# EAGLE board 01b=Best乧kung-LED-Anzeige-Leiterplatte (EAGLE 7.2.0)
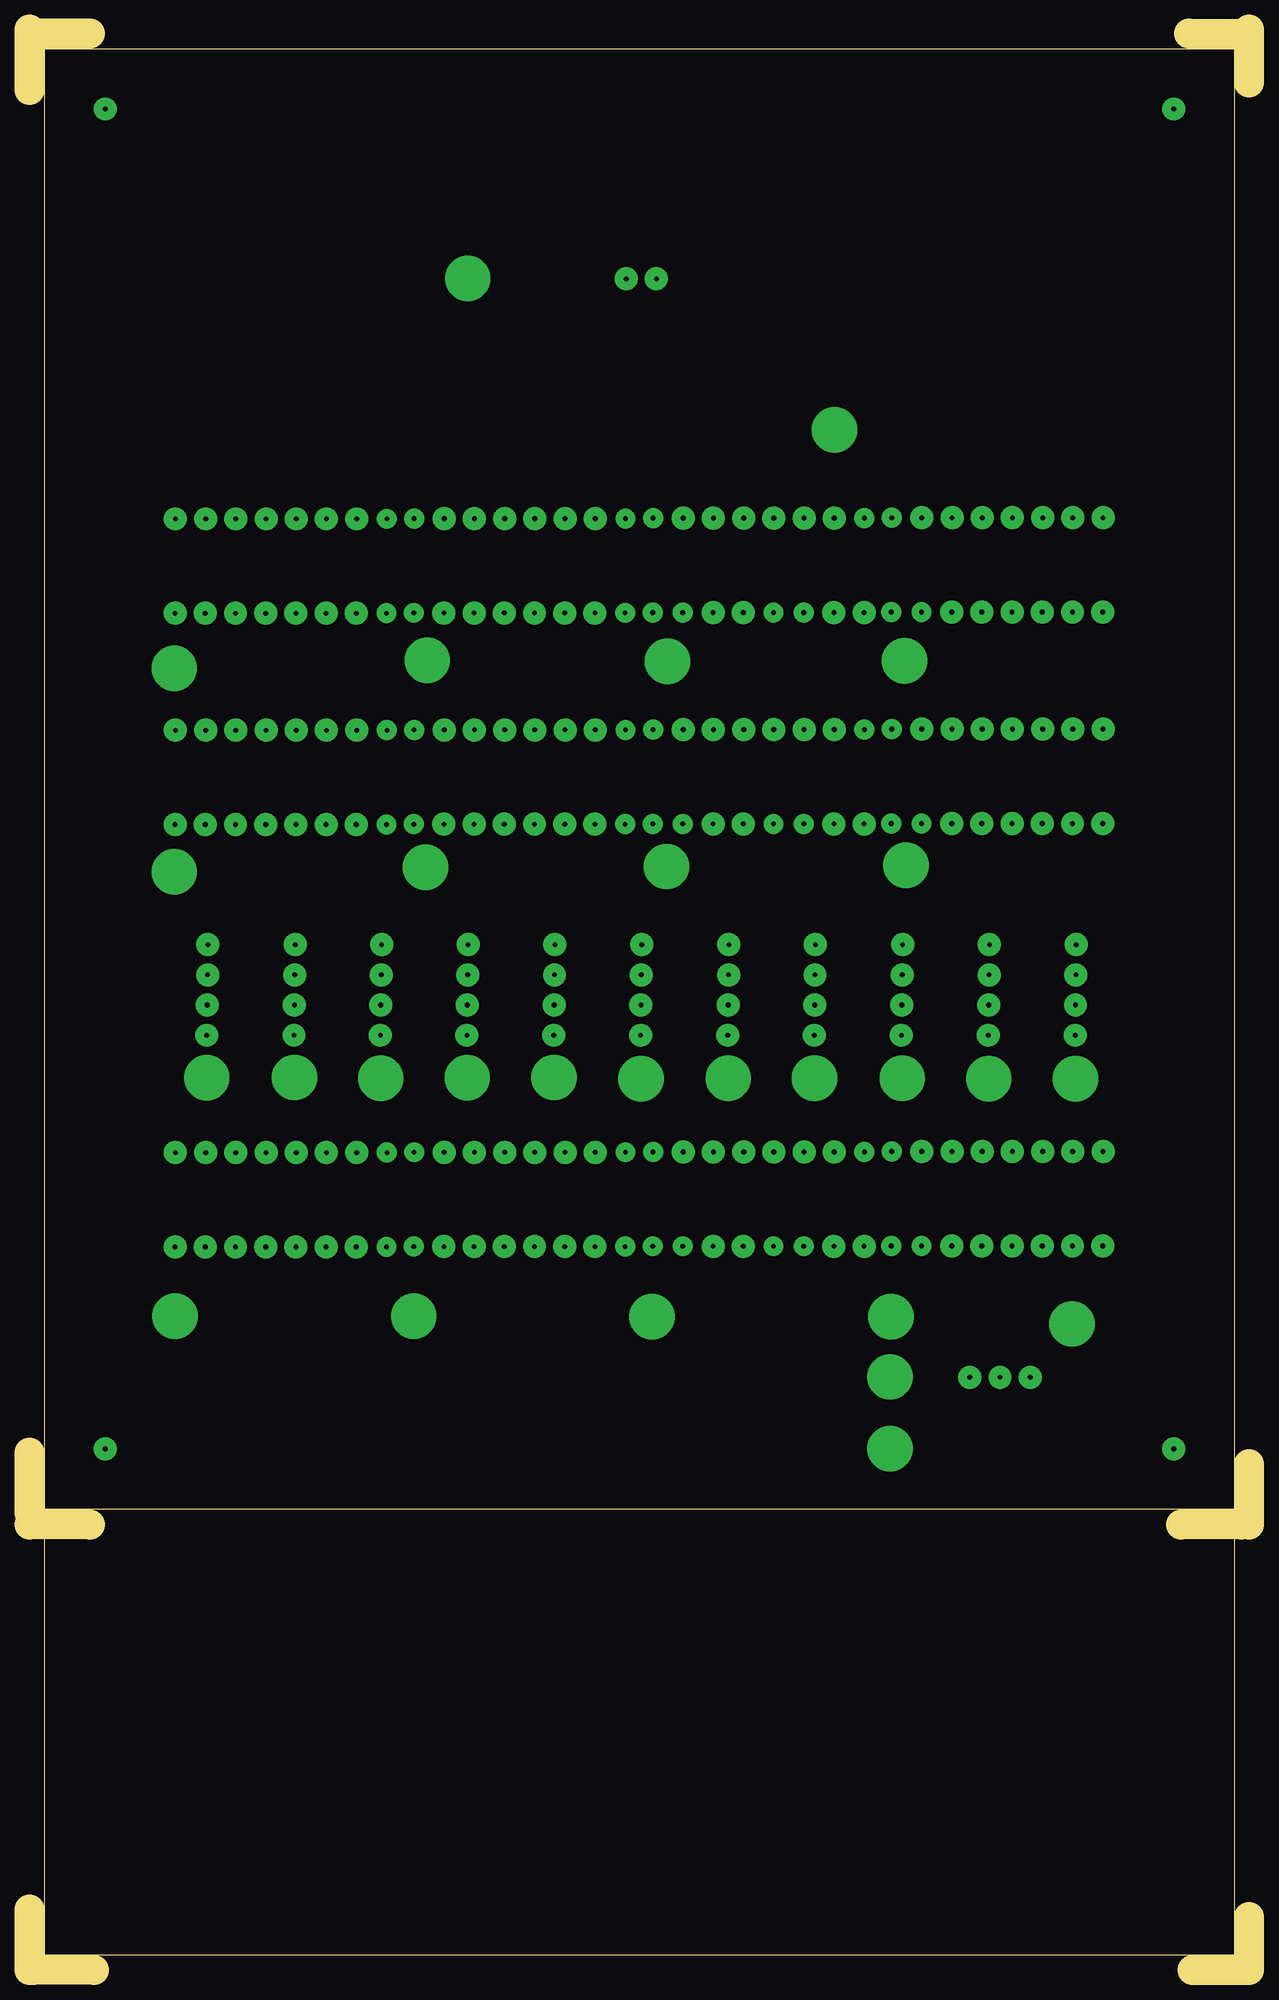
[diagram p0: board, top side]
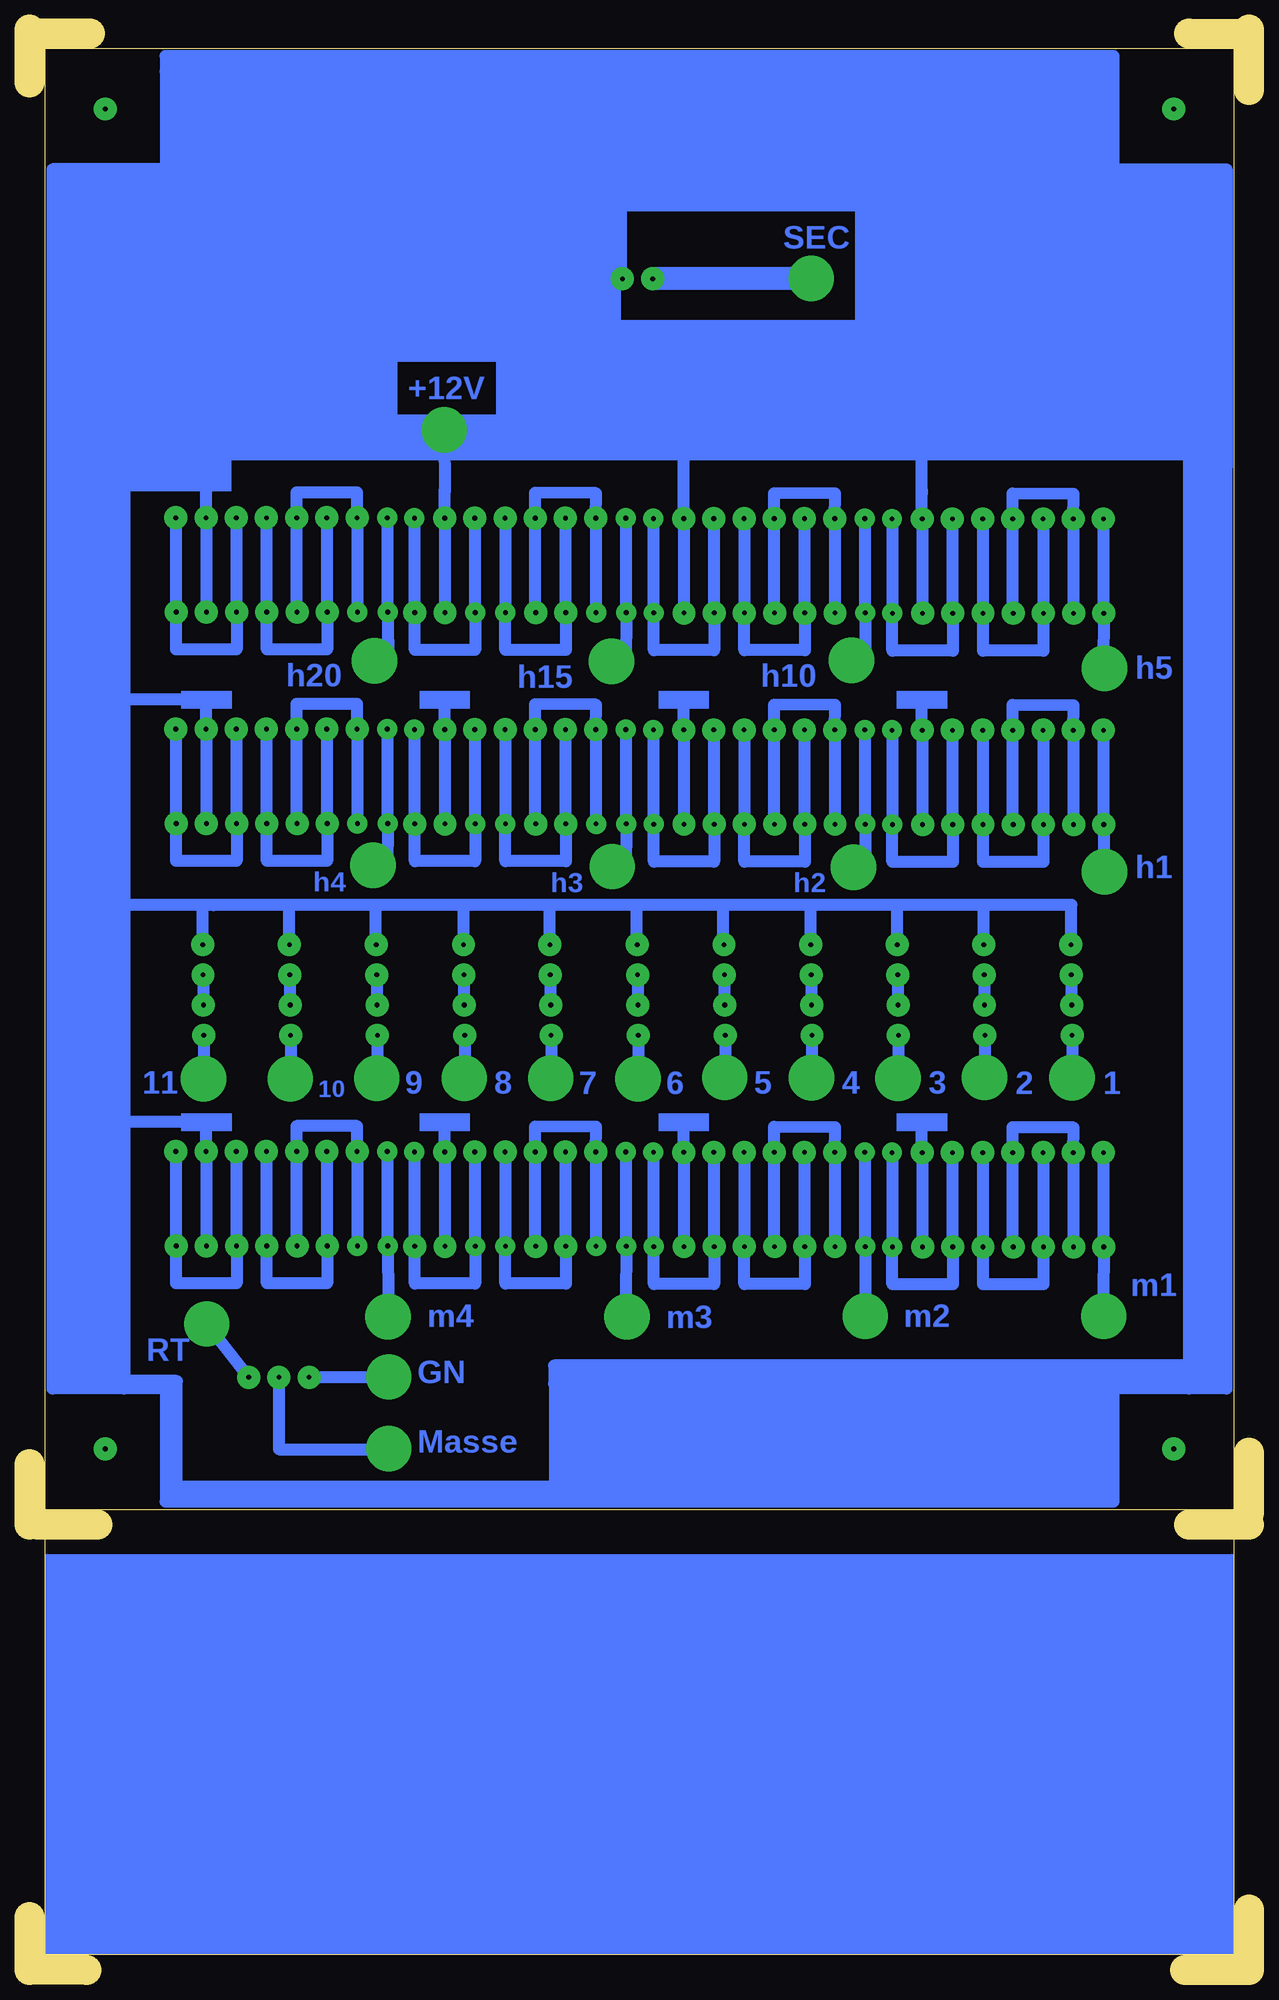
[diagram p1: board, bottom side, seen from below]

Size 102.55 x 163.2 mm. Coordinates in mm from the lower left corner, seen from the top.
Outline: 1.27,38.74 1.27,1.27 101.28,1.27 101.28,38.74
Outline: 1.27,38.74 1.27,161.61 101.28,161.61 101.28,38.74
Outline: 5.4,0 0.32,0
Outline: 0,0 0,5.08
Outline: 97.79,0 102.55,0 102.55,4.45
Outline: 5.08,162.88 0,162.88
Outline: 0,158.12 0,162.88
Outline: 0,162.88 0,163.2
Outline: 102.55,158.75 102.55,163.2
Outline: 97.47,162.88 102.23,162.88
Outline: 101.28,38.74 1.27,38.74
Outline: 0,38.42 0,43.5
Outline: 5.08,37.47 0,37.47
Outline: 101.92,37.47 96.84,37.47
Outline: 102.55,37.47 102.55,42.55
Copper layers (1*16): Top 0.035mm / dielectric 1.5mm / Bottom 0.035mm
Design rules "default": minimum track width 10mil, minimum drill 24mil, track to track 8mil, track to pad 8mil, pad to pad 8mil, via to via 8mil, smd to smd 8mil, copper to edge 40mil, drill to drill 8mil, minimum pad ring 10mil, minimum via ring 8mil, stop-mask expansion 4mil, vias tented up to drill 0mil, thermal gap 10mil

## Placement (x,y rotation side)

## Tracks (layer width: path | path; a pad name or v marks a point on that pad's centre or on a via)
S$1  (via drill 0.4 pad 1.93)
  other vias: 81.6,49.85
S$2  (via drill 0.4 pad 1.93)
  other vias: 96.2,43.82
S$3  (via drill 0 pad 3.81, 0.4 pad 1.93)
  Bottom 1.016: v84.14,49.85 87.63,54.29 v87.66,54.32
S$4  (via drill 0.4 pad 1.93)
  other vias: 6.35,43.82
S$5  (via drill 0 pad 3.81, 0.4 pad 1.93)
  Bottom 1.016: v72.36,49.88 72.39,49.85 v79.06,49.85
  other vias: 72.36,43.85 36.83,142.27 67.69,129.54 33.43,110.14 12.16,109.47 53.63,110.08 73.56,110.11
S$6  (via drill 0.4 pad 1.93)
  other vias: 6.35,156.53
S$7  (via drill 0.4 pad 1.93)
  other vias: 52.71,142.24
S$8  (via drill 0.4 pad 1.93)
  other vias: 50.17,142.24
S$9  (via drill 0.4 pad 1.93)
  other vias: 96.2,156.53
S$10  (via drill 0.4 pad 1.68)
  Bottom 1.016: v32.29,60.83 32.29,56.71
S$11  (via drill 0.4 pad 1.93)
  other vias: 34.83,60.83
S$12  (via drill 0.4 pad 1.93)
  other vias: 42.45,60.83
S$13  (via drill 0.4 pad 1.68, 0.4 pad 1.93)
  Bottom 1.016: v44.99,60.83 44.99,57.69 50.07,57.69 v50.07,60.83
S$14  (via drill 0.4 pad 1.93)
  other vias: 47.53,60.83
S$15  (via drill 0.4 pad 1.68)
  other vias: 32.32,68.77
S$16  (via drill 0.4 pad 1.93)
  Bottom 1.016: 34.86,60.74 v34.86,68.77 34.83,70.87 39.97,70.9 39.97,60.83
S$17  (via drill 0.4 pad 1.93)
  Bottom 1.016: v37.37,60.83 37.37,60.8 | 37.37,60.74 37.37,57.69 42.45,57.69 42.45,60.8 | v37.4,68.77 37.4,60.8 37.37,60.8 | 37.37,60.8 37.37,60.74 | 37.37,60.74 37.43,60.74
S$18  (via drill 0.4 pad 1.93)
  other vias: 39.94,68.77
S$19  (via drill 0.4 pad 1.93)
  Bottom 1.016: v42.48,68.77 42.48,60.8
S$20  (via drill 0.4 pad 1.93)
  Bottom 1.016: v45.02,68.77 45.02,60.8
S$21  (via drill 0.4 pad 1.93)
  Bottom 1.016: v47.56,68.77 47.56,60.8
S$22  (via drill 0.4 pad 1.68)
  Bottom 1.016: v50.1,68.77 50.1,60.83
S$23  (via drill 0.4 pad 1.93)
  other vias: 39.91,60.83
S$24
  Bottom 1.016: 32.32,68.71 32.32,60.83
S$25  (via drill 0.4 pad 1.68)
  Bottom 1.016: v52.39,60.87 52.42,56.39
S$26  (via drill 0.4 pad 1.68)
  other vias: 54.93,60.86
S$27  (via drill 0.4 pad 1.68)
  other vias: 62.55,60.86
S$28  (via drill 0.4 pad 1.68, 0.4 pad 1.93)
  Bottom 1.016: v65.09,60.87 65.09,57.72 70.17,57.72 v70.17,60.87
S$29  (via drill 0.4 pad 1.93)
  other vias: 67.63,60.86
S$30  (via drill 0.4 pad 1.68)
  other vias: 52.42,68.8
S$31  (via drill 0.4 pad 1.93)
  Bottom 1.016: 54.96,60.77 v54.96,68.8 54.93,70.9 60.07,70.93 60.07,60.87
S$32  (via drill 0.4 pad 1.93)
  Bottom 1.016: v57.47,60.87 57.47,60.83 | 57.47,60.77 57.47,57.72 62.55,57.72 62.55,60.83 | v57.5,68.8 57.5,60.83 57.47,60.83 | 57.47,60.83 57.47,60.77 | 57.47,60.77 57.53,60.77
S$33  (via drill 0.4 pad 1.93)
  other vias: 60.04,68.8
S$34  (via drill 0.4 pad 1.93)
  Bottom 1.016: v62.58,68.8 62.58,60.83
S$35  (via drill 0.4 pad 1.93)
  Bottom 1.016: v65.12,68.8 65.12,60.83
S$36  (via drill 0.4 pad 1.93)
  Bottom 1.016: v67.66,68.8 67.66,60.83
S$37  (via drill 0.4 pad 1.68)
  Bottom 1.016: v70.2,68.8 70.2,60.87
S$38  (via drill 0.4 pad 1.93)
  other vias: 60.01,60.86
S$39
  Bottom 1.016: 52.42,68.74 52.42,60.87
S$40  (via drill 0.4 pad 1.68)
  Bottom 1.016: v72.45,60.9 72.42,56.32
S$41  (via drill 0.4 pad 1.68)
  other vias: 74.99,60.9
S$42  (via drill 0.4 pad 1.93)
  other vias: 82.61,60.9
S$43  (via drill 0.4 pad 1.93)
  Bottom 1.016: v85.15,60.9 85.15,57.75 90.23,57.75 v90.23,60.9
S$44  (via drill 0.4 pad 1.93)
  other vias: 87.69,60.9
S$45  (via drill 0.4 pad 1.68)
  other vias: 72.49,68.83
S$46  (via drill 0.4 pad 1.93)
  Bottom 1.016: 75.02,60.8 v75.02,68.83 75.02,70.96 80.14,70.96 80.14,60.9
S$47  (via drill 0.4 pad 1.93)
  Bottom 1.016: v77.53,60.9 77.53,60.87 | 77.53,60.8 77.53,57.75 82.61,57.75 82.61,60.87 | v77.56,68.83 77.56,60.87 77.53,60.87 | 77.53,60.87 77.53,60.8 | 77.53,60.8 77.6,60.8
S$48  (via drill 0.4 pad 1.93)
  other vias: 80.11,68.83
S$49  (via drill 0.4 pad 1.93)
  Bottom 1.016: v82.64,68.83 82.64,60.87
S$50  (via drill 0.4 pad 1.93)
  Bottom 1.016: v85.19,68.83 85.19,60.87
S$51  (via drill 0.4 pad 1.93)
  Bottom 1.016: v87.72,68.83 87.72,60.87
S$52  (via drill 0.4 pad 1.93)
  Bottom 1.016: v90.27,68.83 90.27,60.9
S$53  (via drill 0.4 pad 1.93)
  other vias: 80.07,60.9
S$54
  Bottom 1.016: 72.48,68.77 72.48,60.9
S$55
  Bottom 1.016: 27.53,68.74 27.53,71.12
S$56
  Bottom 1.016: 47.56,68.74 47.56,71.12
S$57
  Bottom 1.016: 67.66,68.74 67.66,71.12
S$58
  Bottom 1.016: 87.69,68.74 87.69,71.12
S$59
  Bottom 1.016: 88.93,71.31 96.01,71.31 96.01,71.34
S$60  (via drill 0.4 pad 1.93)
  Bottom 1.016: v12.22,96.33 12.26,91.92
S$61  (via drill 0.4 pad 1.93)
  other vias: 14.76,96.33
S$62  (via drill 0.4 pad 1.93)
  other vias: 22.38,96.33
S$63  (via drill 0.4 pad 1.68, 0.4 pad 1.93)
  Bottom 1.016: v24.92,96.33 24.92,93.19 30,93.19 v30,96.33
S$64  (via drill 0.4 pad 1.93)
  Bottom 1.016: v12.22,60.8 12.26,56.39
S$65  (via drill 0.4 pad 1.93)
  other vias: 14.76,60.8
S$66  (via drill 0.4 pad 1.93)
  other vias: 22.38,60.8
S$67  (via drill 0.4 pad 1.68, 0.4 pad 1.93)
  Bottom 1.016: v24.92,60.8 24.92,57.66 30,57.66 v30,60.8
S$68  (via drill 0.4 pad 1.93)
  other vias: 27.46,60.8
S$69
  Bottom 1.016: 12.26,68.67 12.26,60.8
S$70  (via drill 0.4 pad 1.93)
  other vias: 12.26,68.74
S$71  (via drill 0.4 pad 1.93)
  Bottom 1.016: 14.79,60.71 v14.79,68.74 14.76,70.83 19.91,70.87 19.91,60.8
S$72  (via drill 0.4 pad 1.93)
  other vias: 19.84,60.8
S$73  (via drill 0.4 pad 1.93)
  other vias: 19.88,68.74
S$74  (via drill 0.4 pad 1.93)
  Bottom 1.016: v22.41,68.74 22.41,60.77
S$75  (via drill 0.4 pad 1.93)
  Bottom 1.016: v24.96,68.74 24.96,60.77
S$76  (via drill 0.4 pad 1.93)
  Bottom 1.016: v27.5,68.74 27.5,60.77
S$77  (via drill 0.4 pad 1.68)
  Bottom 1.016: v30.04,68.74 30.04,60.8
S$78  (via drill 0.4 pad 1.93)
  other vias: 27.46,96.33
S$79  (via drill 0.4 pad 1.93)
  other vias: 12.26,104.27
S$80  (via drill 0.4 pad 1.93)
  Bottom 1.016: 14.79,96.23 v14.79,104.27 14.76,106.36 19.91,106.39 19.91,96.33
S$81  (via drill 0.4 pad 1.93)
  Bottom 1.016: v17.3,60.8 17.3,60.77 | 17.3,60.71 17.3,57.66 22.38,57.66 22.38,60.77 | v17.34,68.74 17.34,60.77 17.3,60.77 | 17.3,60.77 17.3,60.71 | 17.3,60.71 17.37,60.71
S$82  (via drill 0.4 pad 1.93)
  Bottom 1.016: v17.3,96.33 17.3,96.3 | 17.3,96.23 17.3,93.19 22.38,93.19 22.38,96.3 | v17.34,104.27 17.34,96.3 17.3,96.3 | 17.3,96.3 17.3,96.23 | 17.3,96.23 17.37,96.23
S$83  (via drill 0.4 pad 1.93)
  other vias: 19.88,104.27
S$84  (via drill 0.4 pad 1.93)
  Bottom 1.016: v22.41,104.27 22.41,96.3
S$85  (via drill 0.4 pad 1.93)
  Bottom 1.016: v24.96,104.27 24.96,96.3
S$86  (via drill 0.4 pad 1.93)
  Bottom 1.016: v27.5,104.27 27.5,96.3
S$87  (via drill 0.4 pad 1.68)
  Bottom 1.016: v30.04,104.27 30.04,96.33
S$88  (via drill 0.4 pad 1.93)
  other vias: 19.84,96.33
S$89
  Bottom 1.016: 12.26,104.2 12.26,96.33
S$90  (via drill 0.4 pad 1.68)
  Bottom 1.016: v32.29,96.36 32.29,92.23
S$91  (via drill 0.4 pad 1.93)
  other vias: 34.83,96.36
S$92  (via drill 0.4 pad 1.93)
  other vias: 42.45,96.36
S$93  (via drill 0.4 pad 1.68, 0.4 pad 1.93)
  Bottom 1.016: v44.99,96.36 44.99,93.22 50.07,93.22 v50.07,96.36
S$94  (via drill 0.4 pad 1.93)
  other vias: 47.53,96.36
S$95  (via drill 0.4 pad 1.68)
  other vias: 32.32,104.3
S$96  (via drill 0.4 pad 1.93)
  Bottom 1.016: 34.86,96.27 v34.86,104.3 34.83,106.39 39.97,106.43 39.97,96.36
S$97  (via drill 0.4 pad 1.93)
  Bottom 1.016: v37.37,96.36 37.37,96.33 | 37.37,96.27 37.37,93.22 42.45,93.22 42.45,96.33 | v37.4,104.3 37.4,96.33 37.37,96.33 | 37.37,96.33 37.37,96.27 | 37.37,96.27 37.43,96.27
S$98  (via drill 0.4 pad 1.93)
  other vias: 39.94,104.3
S$99  (via drill 0.4 pad 1.93)
  Bottom 1.016: v42.48,104.3 42.48,96.33
S$100  (via drill 0.4 pad 1.93)
  Bottom 1.016: v45.02,104.3 45.02,96.33
S$101  (via drill 0.4 pad 1.93)
  Bottom 1.016: v47.56,104.3 47.56,96.33
S$102  (via drill 0.4 pad 1.68)
  Bottom 1.016: v50.1,104.3 50.1,96.36
S$103  (via drill 0.4 pad 1.93)
  other vias: 39.91,96.36
S$104
  Bottom 1.016: 32.32,104.23 32.32,96.36
S$105  (via drill 0.4 pad 1.68)
  Bottom 1.016: v52.39,96.39 52.42,92.39
S$106  (via drill 0.4 pad 1.68)
  other vias: 54.93,96.39
S$107  (via drill 0.4 pad 1.68)
  other vias: 62.55,96.39
S$108  (via drill 0.4 pad 1.68, 0.4 pad 1.93)
  Bottom 1.016: v65.09,96.39 65.09,93.25 70.17,93.25 v70.17,96.39
S$109  (via drill 0.4 pad 1.93)
  other vias: 67.63,96.39
S$110  (via drill 0.4 pad 1.68)
  other vias: 52.42,104.33
S$111  (via drill 0.4 pad 1.93)
  Bottom 1.016: 54.96,96.3 v54.96,104.33 54.93,106.43 60.07,106.46 60.07,96.39
S$112  (via drill 0.4 pad 1.93)
  Bottom 1.016: v57.47,96.39 57.47,96.36 | 57.47,96.3 57.47,93.25 62.55,93.25 62.55,96.36 | v57.5,104.33 57.5,96.36 57.47,96.36 | 57.47,96.36 57.47,96.3 | 57.47,96.3 57.53,96.3
S$113  (via drill 0.4 pad 1.93)
  other vias: 60.04,104.33
S$114  (via drill 0.4 pad 1.93)
  Bottom 1.016: v62.58,104.33 62.58,96.36
S$115  (via drill 0.4 pad 1.93)
  Bottom 1.016: v65.12,104.33 65.12,96.36
S$116  (via drill 0.4 pad 1.93)
  Bottom 1.016: v67.66,104.33 67.66,96.36
S$117  (via drill 0.4 pad 1.68)
  Bottom 1.016: v70.2,104.33 70.2,96.39
S$118  (via drill 0.4 pad 1.93)
  other vias: 60.01,96.39
S$119
  Bottom 1.016: 52.42,104.27 52.42,96.39
S$120  (via drill 0.4 pad 1.68)
  Bottom 1.016: v72.45,96.42 72.48,92.46
S$121  (via drill 0.4 pad 1.68)
  other vias: 74.99,96.42
S$122  (via drill 0.4 pad 1.93)
  other vias: 82.61,96.42
S$123  (via drill 0.4 pad 1.93)
  Bottom 1.016: v85.15,96.42 85.15,93.28 90.23,93.28 v90.23,96.42
S$124  (via drill 0.4 pad 1.93)
  other vias: 87.69,96.42
S$125  (via drill 0.4 pad 1.68)
  other vias: 72.49,104.36
S$126  (via drill 0.4 pad 1.93)
  Bottom 1.016: 75.02,96.33 v75.02,104.36 75.02,106.49 80.14,106.49 80.14,96.42
S$127  (via drill 0.4 pad 1.93)
  Bottom 1.016: v77.53,96.42 77.53,96.39 | 77.53,96.33 77.53,93.28 82.61,93.28 82.61,96.39 | v77.56,104.36 77.56,96.39 77.53,96.39 | 77.53,96.39 77.53,96.33 | 77.53,96.33 77.6,96.33
S$128  (via drill 0.4 pad 1.93)
  other vias: 80.11,104.36
S$129  (via drill 0.4 pad 1.93)
  Bottom 1.016: v82.64,104.36 82.64,96.39
S$130  (via drill 0.4 pad 1.93)
  Bottom 1.016: v85.19,104.36 85.19,96.39
S$131  (via drill 0.4 pad 1.93)
  Bottom 1.016: v87.72,104.36 87.72,96.39
S$132  (via drill 0.4 pad 1.93)
  Bottom 1.016: v90.27,104.36 90.27,96.42
S$133  (via drill 0.4 pad 1.93)
  other vias: 80.07,96.42
S$134
  Bottom 1.016: 72.48,104.3 72.48,96.42
S$135
  Bottom 1.016: 27.53,104.27 27.53,106.65
S$136
  Bottom 1.016: 47.56,104.27 47.56,106.65
S$137
  Bottom 1.016: 67.66,104.27 67.66,106.65
S$138
  Bottom 1.016: 87.69,104.27 87.69,106.65
S$139
  Bottom 1.016: 88.93,106.84 96.01,106.84
S$140
  Bottom 1.016: 4.98,50.83 58.45,50.83 58.45,49.31
S$141  (via drill 0.4 pad 1.93)
  Bottom 1.016: v12.22,114.11 12.26,109.7
S$142  (via drill 0.4 pad 1.93)
  other vias: 14.76,114.11
S$143  (via drill 0.4 pad 1.93)
  other vias: 22.38,114.11
S$144  (via drill 0.4 pad 1.68, 0.4 pad 1.93)
  Bottom 1.016: v24.92,114.11 24.92,110.97 30,110.97 v30,114.11
S$145  (via drill 0.4 pad 1.93)
  other vias: 27.46,114.11
S$146  (via drill 0.4 pad 1.93)
  other vias: 12.26,122.05
S$147  (via drill 0.4 pad 1.93)
  Bottom 1.016: 14.79,114.01 v14.79,122.05 14.76,124.14 19.91,124.17 19.91,114.11
S$148  (via drill 0.4 pad 1.93)
  Bottom 1.016: v17.3,114.11 17.3,114.08 | 17.3,114.01 17.3,110.97 22.38,110.97 22.38,114.08 | v17.34,122.05 17.34,114.08 17.3,114.08 | 17.3,114.08 17.3,114.01 | 17.3,114.01 17.37,114.01
S$149  (via drill 0.4 pad 1.93)
  other vias: 19.88,122.05
S$150  (via drill 0.4 pad 1.93)
  Bottom 1.016: v22.41,122.05 22.41,114.08
S$151  (via drill 0.4 pad 1.93)
  Bottom 1.016: v24.96,122.05 24.96,114.08
S$152  (via drill 0.4 pad 1.93)
  Bottom 1.016: v27.5,122.05 27.5,114.08
S$153  (via drill 0.4 pad 1.68)
  Bottom 1.016: v30.04,122.05 30.04,114.11
S$154  (via drill 0.4 pad 1.93)
  other vias: 19.84,114.11
S$155
  Bottom 1.016: 12.26,121.98 12.26,114.11
S$156  (via drill 0.4 pad 1.68)
  Bottom 1.016: v32.29,114.14 32.29,110.01
S$157  (via drill 0.4 pad 1.93)
  other vias: 34.83,114.14
S$158  (via drill 0.4 pad 1.93)
  other vias: 42.45,114.14
S$159  (via drill 0.4 pad 1.68, 0.4 pad 1.93)
  Bottom 1.016: v44.99,114.14 44.99,111 50.07,111 v50.07,114.14
S$160  (via drill 0.4 pad 1.93)
  other vias: 47.53,114.14
S$161  (via drill 0.4 pad 1.68)
  other vias: 32.32,122.08
S$162  (via drill 0.4 pad 1.93)
  Bottom 1.016: 34.86,114.05 v34.86,122.08 34.83,124.17 39.97,124.21 39.97,114.14
S$163  (via drill 0.4 pad 1.93)
  Bottom 1.016: v37.37,114.14 37.37,114.11 | 37.37,114.05 37.37,111 42.45,111 42.45,114.11 | v37.4,122.08 37.4,114.11 37.37,114.11 | 37.37,114.11 37.37,114.05 | 37.37,114.05 37.43,114.05
S$164  (via drill 0.4 pad 1.93)
  other vias: 39.94,122.08
S$165  (via drill 0.4 pad 1.93)
  Bottom 1.016: v42.48,122.08 42.48,114.11
S$166  (via drill 0.4 pad 1.93)
  Bottom 1.016: v45.02,122.08 45.02,114.11
S$167  (via drill 0.4 pad 1.93)
  Bottom 1.016: v47.56,122.08 47.56,114.11
S$168  (via drill 0.4 pad 1.68)
  Bottom 1.016: v50.1,122.08 50.1,114.14
S$169  (via drill 0.4 pad 1.93)
  other vias: 39.91,114.14
S$170
  Bottom 1.016: 32.32,122.02 32.32,114.14
S$171  (via drill 0.4 pad 1.68)
  Bottom 1.016: v52.39,114.17 52.42,109.7
S$172  (via drill 0.4 pad 1.68)
  other vias: 54.93,114.17
S$173  (via drill 0.4 pad 1.68)
  other vias: 62.55,114.17
S$174  (via drill 0.4 pad 1.68, 0.4 pad 1.93)
  Bottom 1.016: v65.09,114.17 65.09,111.03 70.17,111.03 v70.17,114.17
S$175  (via drill 0.4 pad 1.93)
  other vias: 67.63,114.17
S$176  (via drill 0.4 pad 1.68)
  other vias: 52.42,122.11
S$177  (via drill 0.4 pad 1.93)
  Bottom 1.016: 54.96,114.08 v54.96,122.11 54.93,124.21 60.07,124.24 60.07,114.17
S$178  (via drill 0.4 pad 1.93)
  Bottom 1.016: v57.47,114.17 57.47,114.14 | 57.47,114.08 57.47,111.03 62.55,111.03 62.55,114.14 | v57.5,122.11 57.5,114.14 57.47,114.14 | 57.47,114.14 57.47,114.08 | 57.47,114.08 57.53,114.08
S$179  (via drill 0.4 pad 1.93)
  other vias: 60.04,122.11
S$180  (via drill 0.4 pad 1.93)
  Bottom 1.016: v62.58,122.11 62.58,114.14
S$181  (via drill 0.4 pad 1.93)
  Bottom 1.016: v65.12,122.11 65.12,114.14
S$182  (via drill 0.4 pad 1.93)
  Bottom 1.016: v67.66,122.11 67.66,114.14
S$183  (via drill 0.4 pad 1.68)
  Bottom 1.016: v70.2,122.11 70.2,114.17
S$184  (via drill 0.4 pad 1.93)
  other vias: 60.01,114.17
S$185
  Bottom 1.016: 52.42,122.05 52.42,114.17
S$186  (via drill 0.4 pad 1.68)
  Bottom 1.016: v72.45,114.2 72.42,109.63
S$187  (via drill 0.4 pad 1.68)
  other vias: 74.99,114.2
S$188  (via drill 0.4 pad 1.93)
  other vias: 82.61,114.2
S$189  (via drill 0.4 pad 1.93)
  Bottom 1.016: v85.15,114.2 85.15,111.06 90.23,111.06 v90.23,114.2
S$190  (via drill 0.4 pad 1.93)
  other vias: 87.69,114.2
S$191  (via drill 0.4 pad 1.68)
  other vias: 72.49,122.14
S$192  (via drill 0.4 pad 1.93)
  Bottom 1.016: 75.02,114.11 v75.02,122.14 75.02,124.27 80.14,124.27 80.14,114.2
S$193  (via drill 0.4 pad 1.93)
  Bottom 1.016: v77.53,114.2 77.53,114.17 | 77.53,114.11 77.53,111.06 82.61,111.06 82.61,114.17 | v77.56,122.14 77.56,114.17 77.53,114.17 | 77.53,114.17 77.53,114.11 | 77.53,114.11 77.6,114.11
S$194  (via drill 0.4 pad 1.93)
  other vias: 80.11,122.14
S$195  (via drill 0.4 pad 1.93)
  Bottom 1.016: v82.64,122.14 82.64,114.17
S$196  (via drill 0.4 pad 1.93)
  Bottom 1.016: v85.19,122.14 85.19,114.17
S$197  (via drill 0.4 pad 1.93)
  Bottom 1.016: v87.72,122.14 87.72,114.17
S$198  (via drill 0.4 pad 1.93)
  Bottom 1.016: v90.27,122.14 90.27,114.2
S$199  (via drill 0.4 pad 1.93)
  other vias: 80.07,114.2
S$200
  Bottom 1.016: 72.48,122.08 72.48,114.2
S$201
  Bottom 1.016: 27.53,122.05 27.53,124.17 27.53,124.43 27.53,128.81
S$202
  Bottom 1.016: 47.56,122.05 47.56,124.43
S$203
  Bottom 1.016: 67.66,122.05 67.66,124.43
S$204
  Bottom 1.016: 87.69,122.05 87.69,124.43
S$205
  Bottom 1.016: 86.14,125.89 96.39,125.79
S$206
  Bottom 1.016: 47.56,124.49 47.56,127.06 47.53,127.06
S$207
  Bottom 1.016: 2.57,126.46 2.57,126.36 2.41,126.36
S$226  (via drill 0.4 pad 1.93)
  other vias: 14.89,78.61
S$227  (via drill 0.4 pad 1.93)
  other vias: 14.92,81.15
S$228  (via drill 0.4 pad 1.93)
  Bottom 1.016: v14.95,83.69 14.95,81.12 14.92,81.12
S$229  (via drill 0.4 pad 1.93)
  other vias: 14.99,86.23
S$230  (via drill 0.4 pad 1.93)
  other vias: 22.22,78.61
S$231  (via drill 0.4 pad 1.93)
  other vias: 22.26,81.15
S$232  (via drill 0.4 pad 1.93)
  Bottom 1.016: v22.29,83.69 22.29,81.12 22.26,81.12
S$233  (via drill 0.4 pad 1.93)
  Bottom 1.016: 14.95,86.23 14.95,89.57 22.32,89.57 | 88.04,86.2 88.04,89.57 22.38,89.57 22.32,89.57 | v22.32,86.23 22.32,89.57
S$234  (via drill 0.4 pad 1.93)
  Bottom 1.016: v29.5,78.61 29.5,74.93
S$235  (via drill 0.4 pad 1.93)
  other vias: 29.53,81.15
S$236  (via drill 0.4 pad 1.93)
  Bottom 1.016: v29.56,83.69 29.56,81.12 29.53,81.12
S$237  (via drill 0.4 pad 1.93)
  Bottom 1.016: v29.59,86.23 29.59,89.44
S$238  (via drill 0.4 pad 1.93)
  other vias: 36.77,78.61
S$239  (via drill 0.4 pad 1.93)
  other vias: 36.8,81.15
S$240  (via drill 0.4 pad 1.93)
  Bottom 1.016: v36.83,83.69 36.83,81.12 36.8,81.12
S$241  (via drill 0.4 pad 1.93)
  other vias: 36.86,86.23
S$242  (via drill 0.4 pad 1.93)
  other vias: 44.07,78.61
S$243  (via drill 0.4 pad 1.93)
  other vias: 44.1,81.15
S$244  (via drill 0.4 pad 1.93)
  Bottom 1.016: v44.13,83.69 44.13,81.12 44.1,81.12
S$245  (via drill 0.4 pad 1.93)
  other vias: 44.16,86.23
S$246  (via drill 0.4 pad 1.93)
  other vias: 51.37,78.61
S$247  (via drill 0.4 pad 1.93)
  other vias: 51.4,81.15
S$248  (via drill 0.4 pad 1.93)
  Bottom 1.016: v51.44,83.69 51.44,81.12 51.4,81.12
S$249  (via drill 0.4 pad 1.93)
  other vias: 51.47,86.23
S$250  (via drill 0.4 pad 1.93)
  other vias: 58.71,78.61
S$251  (via drill 0.4 pad 1.93)
  other vias: 58.74,81.15
S$252  (via drill 0.4 pad 1.93)
  Bottom 1.016: v58.77,83.69 58.77,81.12 58.74,81.12
S$253  (via drill 0.4 pad 1.93)
  other vias: 58.8,86.23
S$254  (via drill 0.4 pad 1.93)
  other vias: 65.98,78.61
S$255  (via drill 0.4 pad 1.93)
  other vias: 66.01,81.15
S$256  (via drill 0.4 pad 1.93)
  Bottom 1.016: v66.04,83.69 66.04,81.12 66.01,81.12
S$257  (via drill 0.4 pad 1.93)
  Bottom 1.016: v66.07,86.23 66.07,89.53
S$258  (via drill 0.4 pad 1.93)
  other vias: 73.31,78.61
S$259  (via drill 0.4 pad 1.93)
  other vias: 73.34,81.15
S$260  (via drill 0.4 pad 1.93)
  Bottom 1.016: v73.37,83.69 73.37,81.12 73.34,81.12
S$261  (via drill 0.4 pad 1.93)
  other vias: 73.41,86.23
S$262  (via drill 0.4 pad 1.93)
  other vias: 80.61,78.61
S$263  (via drill 0.4 pad 1.93)
  other vias: 80.64,81.15
S$264  (via drill 0.4 pad 1.93)
  Bottom 1.016: v80.68,83.69 80.68,81.12 80.64,81.12
S$265  (via drill 0.4 pad 1.93)
  other vias: 80.71,86.23
S$266  (via drill 0.4 pad 1.93)
  other vias: 87.92,78.61
S$267  (via drill 0.4 pad 1.93)
  other vias: 87.95,81.15
S$268  (via drill 0.4 pad 1.93)
  Bottom 1.016: v87.98,83.69 87.98,81.12 87.95,81.12
S$269  (via drill 0.4 pad 1.93)
  other vias: 88.01,86.23
S$270
  Bottom 1.016: 94.58,118.43 94.58,71.63
S$280
  Bottom 1.016: 36.86,86.2 36.86,89.44 36.89,89.44
S$281
  Bottom 1.016: 44.23,86.23 44.23,89.53 44.16,89.53
S$282
  Bottom 1.016: 51.5,86.2 51.5,89.44 51.44,89.44
S$283
  Bottom 1.016: 58.83,86.23 58.83,89.44
S$284
  Bottom 1.016: 73.44,86.23 73.44,89.41 73.5,89.41
S$285
  Bottom 1.016: 80.71,86.27 80.71,89.44
S$286
  Bottom 1.016: 94.58,125.09 94.58,118.46
S$287
  Bottom 1.016: 87.09,89.53 87.09,89.57 94.36,89.57
S$289
  Bottom 1.016: 81.6,49.82 81.6,43.78 72.36,43.78
S$291
  Bottom 1.93: 36.86,142.27 50.17,142.27
S$292
  Bottom 1.016: 67.69,129.35 67.66,124.24
S$297  (via drill 0 pad 3.81)
  other vias: 33.27,92.74 12.16,92.36 53.56,92.81 73.69,92.9 29.53,74.99
S$302  (via drill 0 pad 3.81)
  other vias: 32.29,54.99 12.22,54.99 52.32,54.93 72.42,54.93
S$307
  Bottom 1.016: 22.22,78.68 22.22,74.99
S$308  (via drill 0 pad 3.81)
  other vias: 22.26,75.06
S$309
  Bottom 1.016: 14.86,78.64 14.86,74.96
S$310  (via drill 0 pad 3.81)
  other vias: 14.89,75.03
S$311
  Bottom 1.016: 36.77,78.64 36.77,74.96
S$312  (via drill 0 pad 3.81)
  other vias: 36.8,75.03
S$313
  Bottom 1.016: 44.07,78.68 44.07,74.99
S$314  (via drill 0 pad 3.81)
  other vias: 44.1,75.06
S$315
  Bottom 1.016: 51.37,78.58 51.37,74.9
S$316  (via drill 0 pad 3.81)
  other vias: 51.4,74.96
S$317
  Bottom 1.016: 58.71,78.61 58.71,74.93
S$318  (via drill 0 pad 3.81)
  other vias: 58.74,74.99
S$319
  Bottom 1.016: 65.98,78.61 65.98,74.93
S$320  (via drill 0 pad 3.81)
  other vias: 66.01,74.99
S$321
  Bottom 1.016: 73.34,78.61 73.34,74.93
S$322  (via drill 0 pad 3.81)
  other vias: 73.37,74.99
S$323
  Bottom 1.016: 80.61,78.58 80.61,74.9
S$324  (via drill 0 pad 3.81)
  other vias: 80.64,74.96
S$325
  Bottom 1.016: 87.92,78.58 87.92,74.9
S$326  (via drill 0 pad 3.81)
  other vias: 87.95,74.96
S$327
  Bottom 1.016: 2.35,137.38 99.88,137.19 99.88,137.29
S$329
  Bottom 1.016: 61.82,137.13 61.91,137.13
S$330
  Bottom 1.016: 28.42,151.07 52.86,151.07 52.86,142.08
S$331
  Bottom 1.016: 11.43,156.43 11.43,160.81 28.29,160.81
S$335
  Bottom 1.016: 5.08,48.9 1.91,48.9 1.91,127.95 2.22,127.95 | 5.08,48.9 11.43,48.9 11.43,39.37 58.42,39.37 | 58.42,39.37 91.12,39.37 91.12,48.9 94.61,48.9 | 5.08,127 5.08,48.9 | 58.42,50.45 58.42,40.64 | 58.42,40.64 58.42,39.37 | 94.61,71.75 94.61,49.53 | 94.61,49.53 94.61,48.9 | 94.61,48.9 100.65,48.9 100.65,151.45 91.12,151.45 91.12,159.7 | 91.12,159.7 87.63,159.7 | 91.12,159.7 91.12,160.97 11.43,160.97 11.43,151.45 1.91,151.45 1.91,126.36 | 58.42,40.64 90.17,40.64 90.17,49.53 94.61,49.53
(copper drawn outside any net)
  shapes: Bottom area x43

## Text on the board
Bottom: SEC | +12V | h5 | h10 | h15 | h20 | h1 | h2 | h3 | h4 | 1 | 2 | 3 | 4 | 5 | 6 | 7 | 8 | 9 | 10 | 11 | m1 | m2 | m3 | m4 | RT | GN | Masse
Vias: Auf Bestückungsseite gesehen !
tOrigins: K | Die Bauelemente für | die Bestückung entnehmen | Sie bitte den beiliegenden Datenblättern ! | (die "Einbuchtungen" Halbkreise sind die Markierungen auf den LEDs...) | Leiterplatte: | 1,5mm dick | Cevausit | Alles mit 0,8mm vorbohren ! | Br. | Br. | Br. | Die runden Lötinseln mit der Bezeichnung | NICHT bohren ! | Hier wird auf der Lötseite der Draht (Litze) angelötet. | Die 6stck. (2stck.) Br. Brücken nicht vergessen ! | Br. Brücken mit : | Nur zwischen den Vierecken !!!! Nicht der Leiterzug !!!! | Man muss mitdenken (mit vergleichen zu obigen LEDs) !!!! | Br. | Br. | Br. | K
